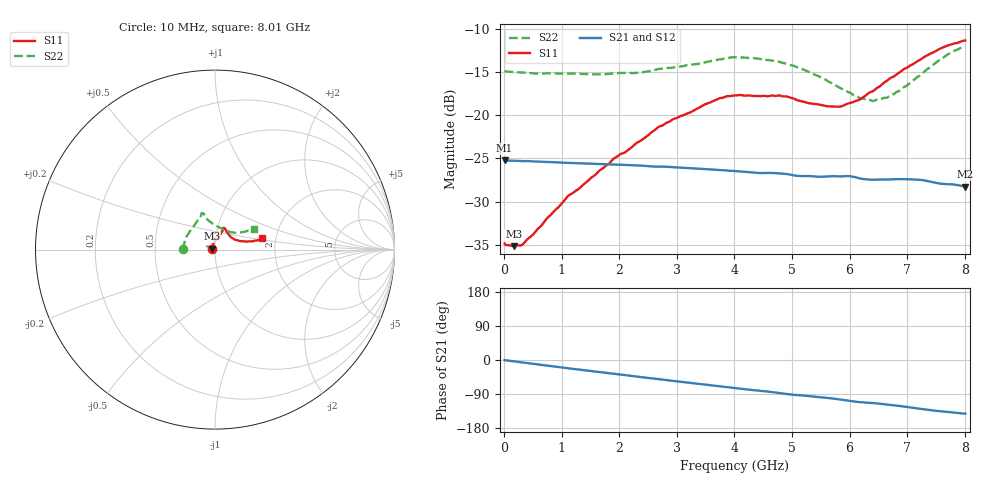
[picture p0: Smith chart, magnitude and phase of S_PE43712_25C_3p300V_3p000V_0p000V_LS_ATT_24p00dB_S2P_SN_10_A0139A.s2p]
! DEVICE ID: PE43712
! File Path: z:\PE43713\PE43713_CHAR_NOM_04292014\AMB\3p300\LS_ATT_24p00dB\PE43713_AMB_3p300V_3p000V_0p000V_LS_ATT_24p00dB_S2P_SN_10_A0139A.s2p
! Serial: 10
! Lot: A0139A
! Temp: 25C
! VDD: 3.300
! VSS: 0.000
! Control_Hi: 3.000
! Control_Lo: 0.000
! Attenuation Step: 24.00dB
! Port 1: RF1
! Port 2: RF2
! ThroughPath:1-2
! IDD: 0.0001450108
! ISS: -1.445e-007
#  Hz  S  RI  R  50
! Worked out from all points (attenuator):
!   801 points, 10 MHz to 8.01 GHz, reference 50 ohm
!   highest |S21| = -25.24 dB at 10 MHz (marker M1); lowest = -28.3 dB at 8.01 GHz (marker M2)
!   lowest |S11| = -35.2 dB at 170 MHz (marker M3), VSWR 1.04, Z = 48.4 + j0.553 ohm
!   |S11| at or under -10 dB: start of sweep to end of sweep
!   |S22| runs from -18.3 to -12.1 dB; largest |S21 - S12| = 0.0002
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1e7  -0.0181 0.000687  0.0547 -0.000256  0.0547 -0.000262  -0.18 0.00119
1.7e8  -0.0165 0.00571  0.0544 -0.00341  0.0545 -0.00341  -0.1776 0.0123
3.3e8  -0.0151 0.00971  0.0539 -0.0065  0.0538 -0.00643  -0.1754 0.0212
1.1e9  -0.0101 0.0322  0.0492 -0.0195  0.0493 -0.0196  -0.1613 0.0659
1.35e9  -0.00643 0.0384  0.0472 -0.0232  0.0472 -0.0233  -0.155 0.0782
1.91e9  0.00508 0.056  0.0417 -0.0307  0.0417 -0.0307  -0.1358 0.1104
2.35e9  0.017 0.0684  0.0364 -0.0359  0.0364 -0.0359  -0.1176 0.1316
2.68e9  0.0272 0.081  0.0322 -0.0387  0.0322 -0.0388  -0.1033 0.1538
3.71e9  0.0448 0.1157  0.0173 -0.045  0.0173 -0.045  -0.0764 0.195
4.01e9  0.0473 0.1214  0.0129 -0.0457  0.0129 -0.0457  -0.0751 0.2035
4.76e9  0.0543 0.1182  0.00249 -0.046  0.00253 -0.046  -0.0601 0.1957
5.35e9  0.0687 0.0943  -0.00484 -0.0441  -0.00482 -0.044  -0.0443 0.1695
5.64e9  0.0801 0.0791  -0.00797 -0.0435  -0.00796 -0.0436  -0.0261 0.1544
5.87e9  0.0909 0.067  -0.0113 -0.0428  -0.0112 -0.0428  -0.00755 0.142
6.16e9  0.1088 0.0564  -0.0155 -0.0403  -0.0154 -0.0403  0.0204 0.1251
6.31e9  0.1219 0.0523  -0.0164 -0.0392  -0.0163 -0.0392  0.0384 0.1163
6.42e9  0.1297 0.05  -0.0171 -0.0388  -0.017 -0.0387  0.0509 0.1099
6.68e9  0.1551 0.0464  -0.0198 -0.0375  -0.0198 -0.0375  0.0819 0.099
7.2e9  0.2022 0.0461  -0.0262 -0.0332  -0.0261 -0.0332  0.1385 0.0957
7.55e9  0.2356 0.0518  -0.0285 -0.0285  -0.0285 -0.0286  0.18 0.1039
7.81e9  0.2537 0.0579  -0.0299 -0.0262  -0.0298 -0.0262  0.2067 0.1128
8.01e9  0.2638 0.0632  -0.0302 -0.024  -0.0301 -0.0241  0.2198 0.1162
